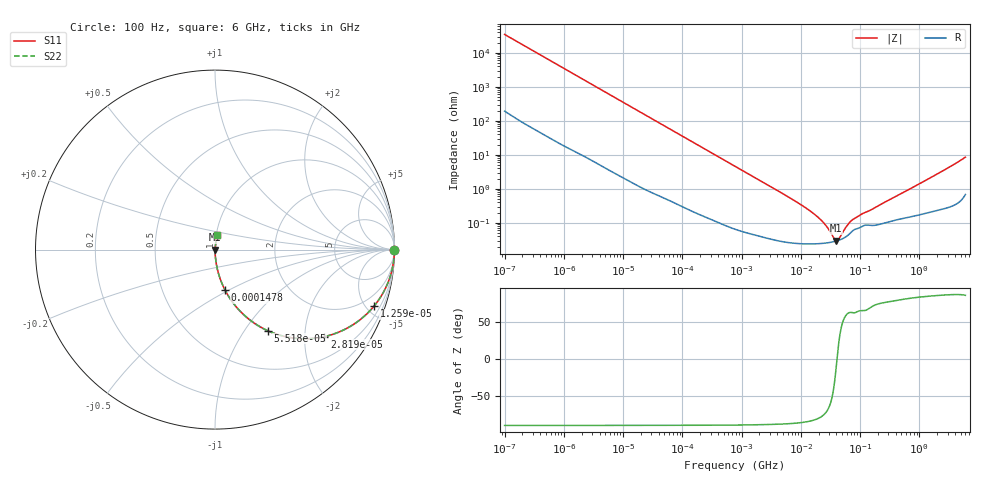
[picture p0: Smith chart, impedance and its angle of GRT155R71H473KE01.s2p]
!Murata Part Number: GRT155R71H473KE01
!These Parameters are Measured in Series Mode Connection
!Data Generated on Jun 19, 2026
!  o--ll--o
!Port1  Port2
!  o------o
!Operation Temp=25[degC], DC Bias Voltage=0[V]
!Freq. Start=100[Hz] Stop=6[GHz] 401[Steps]
# Hz S RI R 50
!Freq.(Hz) S11(Real) S11(Imag) S21(Real) S21(Imag) S12(Real) S12(Imag) S22(Real) S22(Imag)
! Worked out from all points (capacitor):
!   401 points, 100 Hz to 6 GHz, reference 50 ohm
!   read as one part in series: C = 45.9 nF near 109 Hz
!   lowest |Z| = 29.6 mohm at 39.84 MHz (marker M1)
!   series resonance near 40.88 MHz, so ESL is about 330 pH
!   S11 on the Smith chart (normalised r, x): 100 Hz: open; 12.59 kHz: 1.03, -5.59; 28.19 kHz: 1.02, -2.50; 55.18 kHz: 1.01, -1.28; 147.8 kHz: 1.00, -0.48; 6 GHz: 1.01, +0.17
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100  1 -0.00289  2.45e-05 0.00289  2.45e-05 0.00289  1 -0.00289
2008  0.9964 -0.0573  0.00362 0.0573  0.00362 0.0573  0.9964 -0.0573
5378  0.9762 -0.1496  0.0238 0.1496  0.0238 0.1496  0.9762 -0.1496
12592  0.8849 -0.3161  0.1151 0.3161  0.1151 0.3161  0.8849 -0.3161
18841  0.7761 -0.4138  0.2239 0.4138  0.2239 0.4138  0.7761 -0.4138
28191  0.6095 -0.4846  0.3905 0.4846  0.3905 0.4846  0.6095 -0.4846
40335  0.4345 -0.4922  0.5655 0.4922  0.5655 0.4922  0.4345 -0.4922
55182  0.2926 -0.4512  0.7074 0.4512  0.7074 0.4512  0.2926 -0.4512
86348  0.1463 -0.3493  0.8537 0.3493  0.8537 0.3493  0.1463 -0.3493
147774  0.0565 -0.2264  0.9435 0.2264  0.9435 0.2264  0.0565 -0.2264
316350  0.0137 -0.1111  0.9863 0.1111  0.9863 0.1111  0.0137 -0.1111
774597  0.00278 -0.0461  0.9972 0.0461  0.9972 0.0461  0.00278 -0.0461
6353432  0.000292 -0.00559  0.9997 0.00559  0.9997 0.00559  0.000292 -0.00559
1.555665e7  0.000244 -0.002  0.9998 0.002  0.9998 0.002  0.000244 -0.002
2.434276e7  0.000252 -0.000968  0.9997 0.000968  0.9997 0.000968  0.000252 -0.000968
3.64232e7  0.000281 -0.000207  0.9997 0.000207  0.9997 0.000207  0.000281 -0.000207
3.983537e7  0.000293 -4.6e-05  0.9997 4.6e-05  0.9997 4.6e-05  0.000293 -4.6e-05
4.35672e7  0.000307 0.000115  0.9997 -0.000115  0.9997 -0.000115  0.000307 0.000115
5.960426e7  0.000405 0.000695  0.9996 -0.000695  0.9996 -0.000695  0.000405 0.000695
7.455971e7  0.000578 0.00109  0.9994 -0.00109  0.9994 -0.00109  0.000578 0.00109
3.124326e8  0.00111 0.00464  0.9989 -0.00464  0.9989 -0.00464  0.00111 0.00464
6e9  0.0138 0.0834  0.9862 -0.0834  0.9862 -0.0834  0.0138 0.0834
